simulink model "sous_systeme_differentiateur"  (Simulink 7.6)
settings: Solver=ode45  StartTime=0.0  StopTime=10.0  RelTol=1e-3
libraries: fl_lib x6

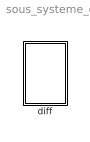
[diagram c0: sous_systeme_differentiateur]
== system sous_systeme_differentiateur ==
  diff : Subsystem

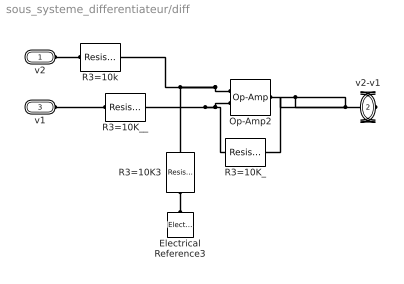
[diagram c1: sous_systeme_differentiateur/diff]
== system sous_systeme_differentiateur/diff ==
  Electrical Reference3 : fl_lib/Electrical/Electrical Elements/Electrical Reference  DialogController=NetworkEngine.DynNeDlgSource  SystemSampleTime=-1  i_Log=off  LocalVarNames=|i  LocalVarDescs=|i  LocalVarLogging=[]
  Op-Amp2 : fl_lib/Electrical/Electrical Elements/Op-Amp  DialogController=NetworkEngine.DynNeDlgSource  SystemSampleTime=-1  i1_Log=off  v1_Log=off  outI_Log=off  LocalVarNames=|i1|v1|outI  LocalVarDescs=|i1|v1|outI  LocalVarLogging=[]
  R3=10K3 : fl_lib/Electrical/Electrical Elements/Resistor  DialogController=NetworkEngine.DynNeDlgSource  SystemSampleTime=-1  R=10e3 Ohm  i_Log=off  v_Log=off  LocalVarNames=|current|voltage|power  LocalVarDescs=|Resistor current (A)|Voltage across resistor (V)|Power (W)  LocalVarLogging=[0 0 0]
  R3=10K_ : fl_lib/Electrical/Electrical Elements/Resistor  DialogController=NetworkEngine.DynNeDlgSource  SystemSampleTime=-1  R=10e3 Ohm  i_Log=off  v_Log=off  LocalVarNames=|current|voltage|power  LocalVarDescs=|Resistor current (A)|Voltage across resistor (V)|Power (W)  LocalVarLogging=[0 0 0]
  R3=10K__ : fl_lib/Electrical/Electrical Elements/Resistor  DialogController=NetworkEngine.DynNeDlgSource  SystemSampleTime=-1  R=10e3 Ohm  i_Log=off  v_Log=off  LocalVarNames=|current|voltage|power  LocalVarDescs=|Resistor current (A)|Voltage across resistor (V)|Power (W)  LocalVarLogging=[0 0 0]
  R3=10k : fl_lib/Electrical/Electrical Elements/Resistor  DialogController=NetworkEngine.DynNeDlgSource  SystemSampleTime=-1  R=10e3 Ohm  i_Log=off  v_Log=off  LocalVarNames=|current|voltage|power  LocalVarDescs=|Resistor current (A)|Voltage across resistor (V)|Power (W)  LocalVarLogging=[0 0 0]
  v2 : PMIOPort  Port=1  Side=Left
  v2-v1 : PMIOPort  Port=2  Side=Right
  v1 : PMIOPort  Port=3  Side=Left
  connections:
  R3=10K3/RConn1 -- Electrical Reference3/LConn1
  Op-Amp2/LConn1 -- R3=10k/RConn1 -- R3=10K3/LConn1
  Op-Amp2/LConn2 -- R3=10K__/RConn1 -- R3=10K_/LConn1
  v2-v1/RConn1 -- R3=10K_/RConn1 -- Op-Amp2/RConn1
  v2/RConn1 -- R3=10k/LConn1
  v1/RConn1 -- R3=10K__/LConn1
